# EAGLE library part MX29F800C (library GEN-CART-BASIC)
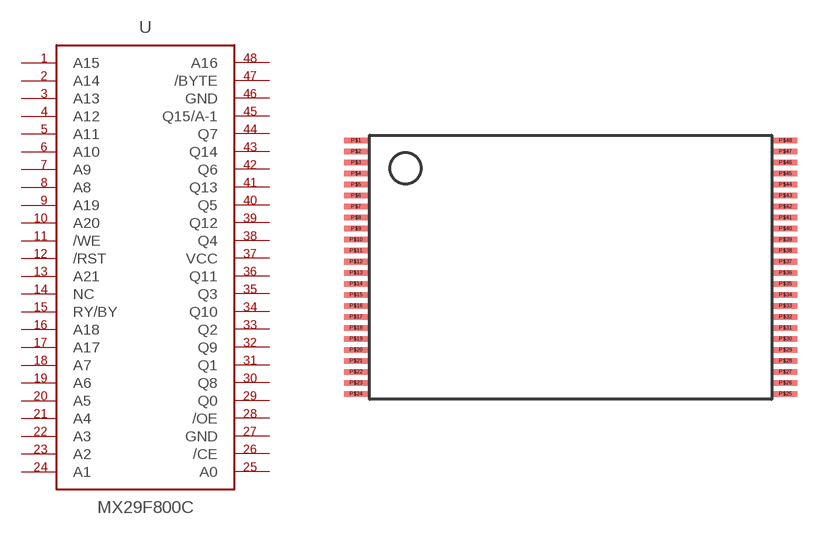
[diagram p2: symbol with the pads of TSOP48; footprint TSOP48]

Designator prefix U

## MX29F800C  [TSOP48]
P$1  A15  in
P$2  A14  in
P$3  A13  in
P$4  A12  in
P$5  A11  in
P$6  A10  in
P$7  A9  in
P$8  A8  in
P$9  A19  in
P$10  A20  in
P$11  /WE  in
P$12  /RST  in
P$13  A21  in
P$14  NC  nc
P$15  RY/BY  out
P$16  A18  in
P$17  A17  in
P$18  A7  in
P$19  A6  in
P$20  A5  in
P$21  A4  in
P$22  A3  in
P$23  A2  in
P$24  A1  in
P$25  A0  in
P$26  /CE  in
P$27  GND  pwr
P$28  /OE  in
P$29  Q0
P$30  Q8
P$31  Q1
P$32  Q9
P$33  Q2
P$34  Q10
P$35  Q3
P$36  Q11
P$37  VCC  pwr
P$38  Q4
P$39  Q12
P$40  Q5
P$41  Q13
P$42  Q6
P$43  Q14
P$44  Q7
P$45  Q15/A-1
P$46  GND  pwr
P$47  /BYTE  in
P$48  A16  in

## Footprint TSOP48 (pad centres in mm)
smd 1.1 x 0.25: P$1 -9.75,5.75; P$2 -9.75,5.25; P$3 -9.75,4.75; P$4 -9.75,4.25; P$5 -9.75,3.75; P$6 -9.75,3.25; P$7 -9.75,2.75; P$8 -9.75,2.25; P$9 -9.75,1.75; P$10 -9.75,1.25; P$11 -9.75,0.75; P$12 -9.75,0.25; P$13 -9.75,-0.25; P$14 -9.75,-0.75; P$15 -9.75,-1.25; P$16 -9.75,-1.75; P$17 -9.75,-2.25; P$18 -9.75,-2.75; P$19 -9.75,-3.25; P$20 -9.75,-3.75; P$21 -9.75,-4.25; P$22 -9.75,-4.75; P$23 -9.75,-5.25; P$24 -9.75,-5.75; P$25 9.75,-5.75; P$26 9.75,-5.25; P$27 9.75,-4.75; P$28 9.75,-4.25; P$29 9.75,-3.75; P$30 9.75,-3.25; P$31 9.75,-2.75; P$32 9.75,-2.25; P$33 9.75,-1.75; P$34 9.75,-1.25; P$35 9.75,-0.75; P$36 9.75,-0.25; P$37 9.75,0.25; P$38 9.75,0.75; P$39 9.75,1.25; P$40 9.75,1.75; P$41 9.75,2.25; P$42 9.75,2.75; P$43 9.75,3.25; P$44 9.75,3.75; P$45 9.75,4.25; P$46 9.75,4.75; P$47 9.75,5.25; P$48 9.75,5.75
